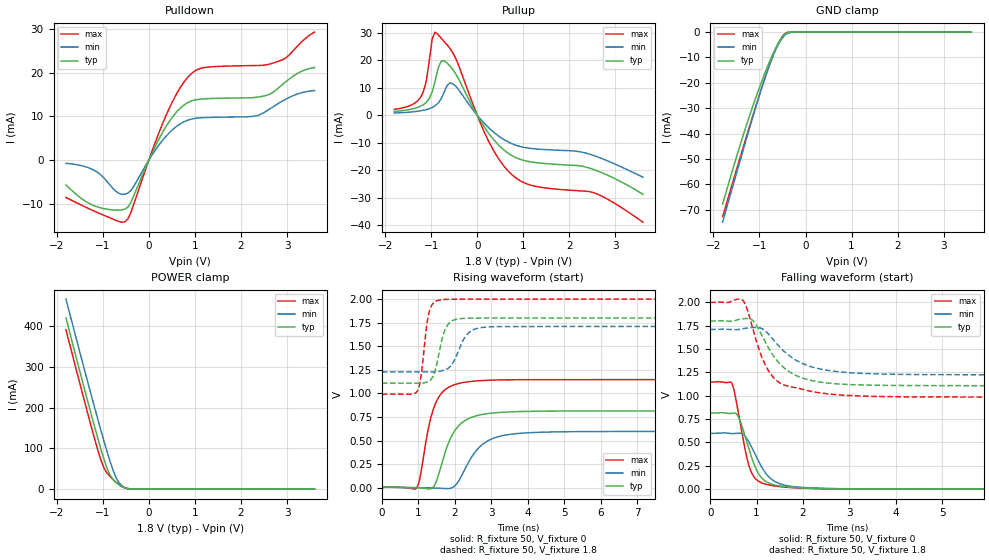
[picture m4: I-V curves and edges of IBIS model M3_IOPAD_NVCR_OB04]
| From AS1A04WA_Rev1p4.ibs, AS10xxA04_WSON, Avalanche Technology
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[Model] M3_IOPAD_NVCR_OB04
Model_type I/O
Enable   Active-High
Vinl  =  0.54
Vinh  =  1.26
Vmeas =  0.9
Cref  =  30e-12
| Capacitance  typ   min   max
C_comp   3.869840e-12   3.575244e-12   4.229518e-12
| Variables   typ   min   max
[GND Clamp Reference]   0   0   0
[POWER Clamp Reference]   1.8   1.71   2
[Pulldown Reference]   0   0   0
[Pullup Reference]   1.8   1.71   2
[Temperature Range]   25   125   -40
[Voltage Range]   1.8   1.71   2
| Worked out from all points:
|   slope of the pulldown table from 0 to 0.27 V, typ, clamps not added: 46.6 ohm
|   slope of the pullup table from 0 to 0.27 V, typ, clamps not added: 38.6 ohm
|   GND clamp passes 1 mA (typ) near -0.46 V on its own axis
|   POWER clamp passes 1 mA (typ) near -0.44 V on its own axis
|   falling waveform, R_fixture 50, V_fixture 0: 20-80 % time 347ps typ, 425ps min, 280ps max; typ from 0.814 V to 0 V
|   falling waveform, R_fixture 50, V_fixture 1.8: 20-80 % time 649ps typ, 775ps min, 500ps max; typ from 1.8 V to 1.1 V
|   rising waveform, R_fixture 50, V_fixture 0: 20-80 % time 520ps typ, 650ps min, 397ps max; typ from 0 V to 0.814 V
|   rising waveform, R_fixture 50, V_fixture 1.8: 20-80 % time 256ps typ, 366ps min, 184ps max; typ from 1.1 V to 1.8 V
[GND Clamp]
| Voltage   I(typ)   I(min)   I(max)
-1.8V     -67.84mA   -74.98mA   -72.81mA
-1.499V   -49.26mA   -55.7mA    -54.28mA
-1.303V   -37.87mA   -43.36mA   -42.4mA
-1.043V   -23.96mA   -27.4mA    -27.1mA
-847.2mV  -14.58mA   -16.27mA   -16.36mA
-716.9mV  -8.973mA   -9.798mA   -9.837mA
-651.7mV  -6.447mA   -7.048mA   -6.896mA
-521.4mV  -2.255mA   -2.801mA   -2.141mA
-456.2mV  -849.3uA   -1.361mA   -679.4uA
-391mV    -172uA     -473.2uA   -88.88uA
-260.7mV  -2.088uA   -22.04uA   -254.3nA
3.6V      0A         0A         0A
[POWER Clamp]
| Voltage   I(typ)   I(min)   I(max)
-1.8V     419.8mA    466.1mA    390.9mA
-1.303V   205.4mA    252.8mA    175.7mA
-1.043V   98.85mA    144.9mA    72.14mA
-977.6mV  74.56mA    119mA      52.56mA
-912.4mV  52.76mA    93.87mA    40.16mA
-847.2mV  35.48mA    69.92mA    31.71mA
-716.9mV  16.42mA    29.44mA    17.31mA
-651.7mV  10.9mA     16.21mA    11.28mA
-586.6mV  6.514mA    8.5mA      6.386mA
-456.2mV  1.168mA    1.854mA    921.1uA
-325.9mV  31.2uA     159.5uA    13.68uA
3.6V      0A         0A         0A
[Pulldown]
| Voltage   I(typ)   I(min)   I(max)
-1.8V     -5.69mA    -732.8uA   -8.548mA
-1.173V   -10.5mA    -2.407mA   -11.73mA
-716.9mV  -11.43mA   -7.123mA   -13.76mA
-521.4mV  -11.21mA   -7.798mA   -14.11mA
-391mV    -9.672mA   -6.953mA   -11.98mA
372.4mV   7.658mA    5.437mA    10.17mA
869mV     13.26mA    9.198mA    19.2mA
1.179V    13.97mA    9.684mA    21.08mA
2.283V    14.28mA    10.02mA    21.59mA
2.766V    16.04mA    12.62mA    22.39mA
3.248V    19.92mA    15.17mA    26.27mA
3.6V      21.15mA    15.89mA    29.24mA
[Pullup]
| Voltage   I(typ)   I(min)   I(max)
-1.8V     1.352mA    789.5uA    2.099mA
-1.238V   3.177mA    1.572mA    6.26mA
-1.108V   4.622mA    2.015mA    12.15mA
-977.6mV  8.411mA    2.79mA     27.68mA
-912.4mV  12.48mA    3.432mA    30.16mA
-782.1mV  19.57mA    5.979mA    27.92mA
-521.4mV  16.37mA    11.35mA    22.45mA
186.2mV   -5.049mA   -3.49mA    -7.284mA
744.8mV   -14.56mA   -10.25mA   -21.44mA
1.241V    -17.12mA   -12.19mA   -25.69mA
2.559V    -19.89mA   -14.78mA   -28.27mA
3.6V      -28.69mA   -22.5mA    -38.81mA
[Ramp]
dV/dt_r   0.488568/0.519945n  0.3582/0.649804n  0.687926/0.397312n
dV/dt_f   0.417076/0.649039n  0.291154/0.774597n  0.608145/0.500349n
R_load = 50
[Falling Waveform]
R_fixture = 50
V_fixture = 0
V_fixture_min = 0
V_fixture_max = 0
| Time   V(typ)   V(min)   V(max)
0s        814.3mV    597mV      1.147V
474.1ps   813.8mV    595.5mV    1.125V
599.7ps   783.2mV    599.8mV    837.3mV
776.9ps   525.9mV    551.6mV    365.8mV
857.5ps   394.6mV    485.8mV    218.7mV
948.2ps   264.1mV    396.3mV    129.1mV
1.169ns   92.84mV    190.4mV    56.83mV
1.546ns   30.54mV    50.91mV    24.51mV
3.59ns    987.2uV    1.63mV     780.3uV
21.88ns   242.1nV    1.102uV    249.8nV
[Falling Waveform]
R_fixture = 50
V_fixture = 1.8
V_fixture_min = 1.71
V_fixture_max = 2
| Time   V(typ)   V(min)   V(max)
0s        1.8V       1.71V      2V
684.9ps   1.824V     1.717V     2.031V
791.9ps   1.828V     1.726V     1.935V
954.3ps   1.787V     1.732V     1.656V
1.128ns   1.633V     1.716V     1.397V
1.355ns   1.433V     1.605V     1.2V
1.831ns   1.222V     1.387V     1.089V
2.549ns   1.136V     1.271V     1.02V
4.583ns   1.109V     1.227V     987.9mV
21.88ns   1.105V     1.225V     986.4mV
[Rising Waveform]
R_fixture = 50
V_fixture = 0
V_fixture_min = 0
V_fixture_max = 0
| Time   V(typ)   V(min)   V(max)
0s        74.44nV    863.5nV    131.9nV
944.2ps   468.1uV    1.924mV    -6.144mV
1.049ns   -1.961mV   1.531mV    113mV
1.314ns   -12.28mV   -427.4uV   697.4mV
1.509ns   84.57mV    -3.045mV   925.6mV
1.949ns   574.2mV    5.58mV     1.087V
2.418ns   740.7mV    298.7mV    1.126V
3.009ns   791.1mV    517.2mV    1.141V
4.315ns   811.6mV    588.4mV    1.146V
21.88ns   814.3mV    597mV      1.147V
[Rising Waveform]
R_fixture = 50
V_fixture = 1.8
V_fixture_min = 1.71
V_fixture_max = 2
| Time   V(typ)   V(min)   V(max)
0s        1.105V     1.225V     986.4mV
973.3ps   1.108V     1.227V     1.024V
1.065ns   1.109V     1.226V     1.158V
1.296ns   1.131V     1.227V     1.861V
1.443ns   1.219V     1.229V     1.968V
1.614ns   1.514V     1.237V     1.992V
1.902ns   1.764V     1.297V     1.998V
2.365ns   1.797V     1.637V     1.999V
2.86ns    1.799V     1.703V     1.999V
21.88ns   1.8V       1.71V      2V
